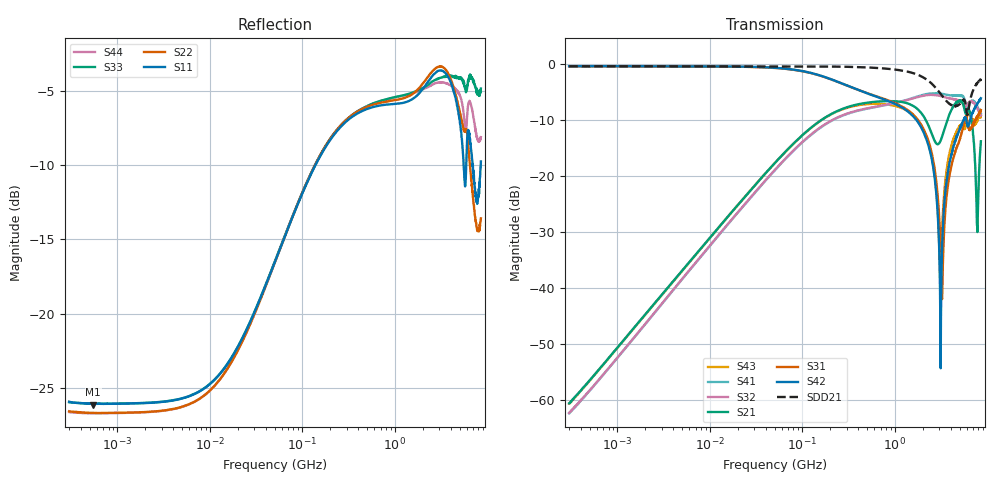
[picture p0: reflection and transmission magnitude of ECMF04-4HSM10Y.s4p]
!ECMF04-4HSM10Y
!Typical device
!Probes on pads
!Port 1: IN1
!Port 2: IN2
!Port 3: OUT1
!Port 4: OUT2
!P1 Probe Type :ACP40-SSG-500; Probe S/N : F628M
!P2 Probe Type :ACP40-SSG-500; Probe S/N : F628M
!P3 Probe Type :ACP40-GSS-500; Probe S/N : DF28F
!P4 Probe Type :ACP40-GSS-500; Probe S/N : DF28F
!Instrument Manufacturer: Agilent Technologies
!Instrument Model: E5071B
!Instrument Serial Number: MY42301810
!Instrument Firmware Rev: A.08.11
!Start Freq. :300.000kHz; Stop Freq. : 8.500GHz
!Number of points : 1601; Sweep : LOGARITHMIC
!Ports power : 0.000000dBm; IFBW : 100.000000Hz
!Calibration kit : 129-248 (9079)
!Prober : PM8 (Manual prober)
!Darkness measurement :YES
!Voltage measurement :NO
!Temperature measurement :NO
!Lane #1 or Lane #2
! Freq ReS11 ImS11 ReS12 ImS12 ReS13 ImS13 ReS14 ImS14
!  ReS21 ImS21 ReS22 ImS22 ReS23 ImS23 ReS24 ImS24
!  ReS31 ImS31 ReS32 ImS32 ReS33 ImS33 ReS34 ImS34
!  ReS41 ImS41 ReS42 ImS42 ReS43 ImS43 ReS44 ImS44
# Hz  S  RI  R  50
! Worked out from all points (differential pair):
!   1601 points, 300 kHz to 8.5 GHz, reference 50 ohm
!   strongest paths, dB at 300 kHz, 3.892 MHz, 50.5 MHz, 655.2 MHz, 8.5 GHz:
!     S42: -0.4, -0.4, -0.7, -5.9, -6.1
!     S31: -0.4, -0.4, -0.7, -5.9, -8.2
!     S21: -60.5, -39.0, -17.6, -6.7, -13.8
!     S32: -62.3, -40.5, -18.9, -7.6, -9.2
!     S41: -62.3, -40.6, -18.9, -7.6, -8.9
!     S43: -60.6, -39.0, -17.6, -7.1, -9.0
!   taken as a pair (ports 2,1 in; 4,3 out), SDD21 dB: -0.4, -0.4, -0.4, -0.7, -2.7
!   lowest |S11| = -26.1 dB at 547.1 kHz (marker M1), VSWR 1.10, Z = 55.2 + j0.163 ohm
!   |S11| at or under -10 dB: start of sweep to 138.5 MHz; 5.526 GHz to 5.904 GHz (377.7 MHz wide, 6.61 % of centre); 6.962 GHz to 8.473 GHz (1.51 GHz wide, 19.6 % of centre)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
300000  0.0507 0.000657  0.000228 0.000914  0.9504 -0.000737  -0.000229 -0.000738
        0.00023 0.000912  0.0471 0.000548  -0.000228 -0.000726  0.954 -0.000809
        0.9503 -0.00103  -0.000222 -0.000737  0.0504 0.000702  0.000235 0.000908
        -0.00023 -0.000731  0.9527 -0.00135  0.000238 0.000903  0.0467 0.000534
547061.6  0.0496 0.00148  0.000249 0.00163  0.95 -0.00141  -0.000224 -0.00131
          0.000252 0.00162  0.0465 0.00131  -0.000233 -0.00131  0.9532 -0.000958
          0.9492 -0.000103  -0.000226 -0.00132  0.0497 0.00121  0.000244 0.00161
          -0.000231 -0.00131  0.9541 -0.00164  0.000253 0.00161  0.0464 0.00141
2.749674e8  0.3865 0.1943  0.3465 0.1986  0.5858 -0.3079  -0.3342 -0.0959
            0.3456 0.1995  0.3893 0.1997  -0.3345 -0.1001  0.5839 -0.3133
            0.586 -0.308  -0.3354 -0.0993  0.4045 0.167  0.3562 0.1721
            -0.3338 -0.0958  0.5838 -0.3129  0.3557 0.1724  0.405 0.165
1.970531e9  0.5465 -0.1472  0.3132 -0.1573  0.0829 -0.2673  0.1333 0.509
            0.3202 -0.1568  0.5631 -0.1741  0.1195 0.5095  0.0774 -0.2521
            0.0761 -0.2665  0.1282 0.5013  0.3312 -0.4671  0.1687 -0.2101
            0.1366 0.5093  0.0697 -0.2516  0.1705 -0.212  0.3098 -0.4741
3.125852e9  0.4482 -0.4798  0.2005 0.0285  -0.0103 -0.0251  0.4947 0.2314
            0.2054 0.0299  0.4376 -0.5171  0.4854 0.2276  0.00653 -0.0109
            -0.0144 -0.0141  0.4688 0.2188  -0.0971 -0.6128  0.0122 0.00523
            0.4935 0.2297  0.000404 0.00189  0.0123 0.00578  -0.0949 -0.5901
3.986114e9  0.1341 -0.5863  0.3433 0.0848  0.066 0.0702  0.5303 -0.0209
            0.3618 0.0875  0.1227 -0.6038  0.5103 -0.035  0.0914 0.0808
            0.0723 0.0878  0.4905 -0.0185  -0.4198 -0.4671  0.0851 0.1342
            0.524 -0.0208  0.1047 0.0986  0.0914 0.1463  -0.3727 -0.451
8.5e9  -0.3232 -0.034  0.0686 0.201  0.4037 -0.1565  -0.3283 -0.1563
       0.0762 0.1896  -0.2086 -0.0157  -0.2901 -0.0561  0.442 -0.2479
       0.3787 -0.0804  -0.3142 -0.145  -0.3117 0.4787  0.3288 0.164
       -0.3297 -0.1373  0.4406 -0.2244  0.3485 0.0603  -0.312 0.2377
